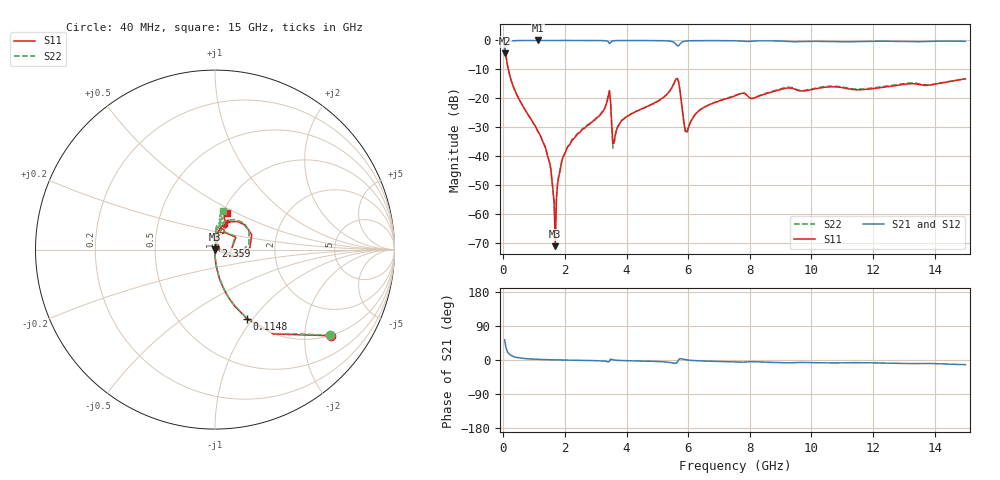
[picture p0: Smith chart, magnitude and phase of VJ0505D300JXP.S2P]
! VJ0505D300JXP
! MLCC placed on 25 mil thick microstrip substrate in series configuraton.
! DATE 06/29/2018  09:14
! CORRECTED  DATA
# GHz  S  MA  R  50.00
!  FREQ  S11M  S11A  S21M  S21A  S12M  S12A  S22M  S22A
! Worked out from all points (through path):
!   401 points, 40 MHz to 15 GHz, reference 50 ohm
!   highest |S21| = -0.01 dB at 1.125 GHz (marker M1); lowest = -4.5 dB at 40 MHz (marker M2)
!   group delay of S21, straight-line fit = 2.92 ps
!   lowest |S11| = -71.1 dB at 1.686 GHz (marker M3), VSWR 1.00, Z = 50 - j0.0184 ohm
!   |S11| at or under -10 dB: 161.3 MHz to end of sweep
!   |S22| runs from -65.5 to -2.0 dB; largest |S21 - S12| = 0.0026
!   S11 on the Smith chart (normalised r, x): 40 MHz: 0.99, -2.70; 114.8 MHz: 0.99, -0.94; 2.359 GHz: 1.00, +0.04; 15 GHz: 1.04, +0.45
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0.04  0.8048 -36.6  0.5957 53.4  0.5963 53.4  0.7981 -36.6
0.1148  0.4246 -65.2  0.905 25.1  0.906 25.1  0.4207 -65.1
0.414  0.1222 -83.5  0.9916 7.0  0.9919 7.1  0.1211 -83.2
1.1246  0.02661 -90.1  0.9985 1.8  0.9989 1.9  0.02641 -90.2
1.4612  0.009096 -91.0  0.9982 0.8  0.9985 0.9  0.008984 -94.5
1.5734  0.004066 -90.2  0.9982 0.6  0.9988 0.7  0.004053 -97.6
1.6108  0.002565 -87.1  0.998 0.5  0.9986 0.6  0.002475 -104.6
1.6856  0.000278 -41.4  0.9984 0.3  0.9985 0.4  0.0005311 -175.9
1.9474  0.009897 85.6  0.997 -0.1  0.9976 -0.1  0.01009 92.8
2.3588  0.02233 85.8  0.9965 -0.7  0.9973 -0.6  0.0229 90.2
2.5458  0.02822 85.9  0.9965 -1.0  0.997 -0.9  0.02901 89.7
3.406  0.1105 60.6  0.9497 -5.0  0.9505 -5.0  0.1117 64.2
3.6304  0.02271 70.3  0.992 -0.4  0.9925 -0.3  0.02248 80.2
3.9296  0.04473 82.8  0.9953 -1.6  0.996 -1.6  0.04481 90.5
5.0516  0.0919 80.6  0.9906 -4.1  0.991 -4.0  0.09071 87.6
5.65  0.2206 22.0  0.8044 -5.1  0.805 -5.1  0.2168 28.6
5.9492  0.02653 35.3  0.9782 0.3  0.9784 0.4  0.0249 45.1
6.4354  0.06565 79.7  0.9916 -2.5  0.9925 -2.4  0.06561 89.3
7.52  0.1108 77.1  0.9851 -5.1  0.9862 -5.1  0.1126 86.5
10.0258  0.142 70.5  0.9658 -7.0  0.9675 -7.0  0.146 78.5
12.5316  0.1598 69.5  0.9678 -8.5  0.9686 -8.5  0.165 80.7
15  0.2166 71.9  0.9644 -12.3  0.965 -12.3  0.2173 77.9
